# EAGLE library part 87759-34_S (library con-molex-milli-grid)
HEADER
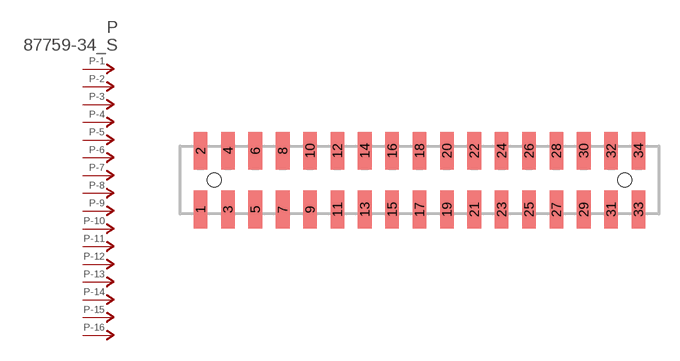
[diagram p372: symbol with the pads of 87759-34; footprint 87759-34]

Designator prefix P; gates -1=P-NV -2=P-N -3=P-N -4=P-N -5=P-N -6=P-N -7=P-N -8=P-N -9=P-N -10=P-N -11=P-N -12=P-N -13=P-N -14=P-N -15=P-N -16=P-N -17=P-N -18=P-N -19=P-N -20=P-N -21=P-N -22=P-N -23=P-N -24=P-N -25=P-N -26=P-N -27=P-N -28=P-N -29=P-N -30=P-N -31=P-N -32=P-N -33=P-N -34=P-N

## 87759-34_S  [87759-34]
1  -1:P  pas
2  -2:P  pas
3  -3:P  pas
4  -4:P  pas
5  -5:P  pas
6  -6:P  pas
7  -7:P  pas
8  -8:P  pas
9  -9:P  pas
10  -10:P  pas
11  -11:P  pas
12  -12:P  pas
13  -13:P  pas
14  -14:P  pas
15  -15:P  pas
16  -16:P  pas
17  -17:P  pas
18  -18:P  pas
19  -19:P  pas
20  -20:P  pas
21  -21:P  pas
22  -22:P  pas
23  -23:P  pas
24  -24:P  pas
25  -25:P  pas
26  -26:P  pas
27  -27:P  pas
28  -28:P  pas
29  -29:P  pas
30  -30:P  pas
31  -31:P  pas
32  -32:P  pas
33  -33:P  pas
34  -34:P  pas

## Footprint 87759-34 (pad centres in mm)
HEADER SMD Dual Row, Vertical
smd 1 x 2.75: 1 -16,-2.15; 2 -16,2.15; 3 -14,-2.15; 4 -14,2.15; 5 -12,-2.15; 6 -12,2.15; 7 -10,-2.15; 8 -10,2.15; 9 -8,-2.15; 10 -8,2.15; 11 -6,-2.15; 12 -6,2.15; 13 -4,-2.15; 14 -4,2.15; 15 -2,-2.15; 16 -2,2.15; 17 0,-2.15; 18 0,2.15; 19 2,-2.15; 20 2,2.15; 21 4,-2.15; 22 4,2.15; 23 6,-2.15; 24 6,2.15; 25 8,-2.15; 26 8,2.15; 27 10,-2.15; 28 10,2.15; 29 12,-2.15; 30 12,2.15; 31 14,-2.15; 32 14,2.15; 33 16,-2.15; 34 16,2.15
hole 1 at -15,0
hole 1 at 15,0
